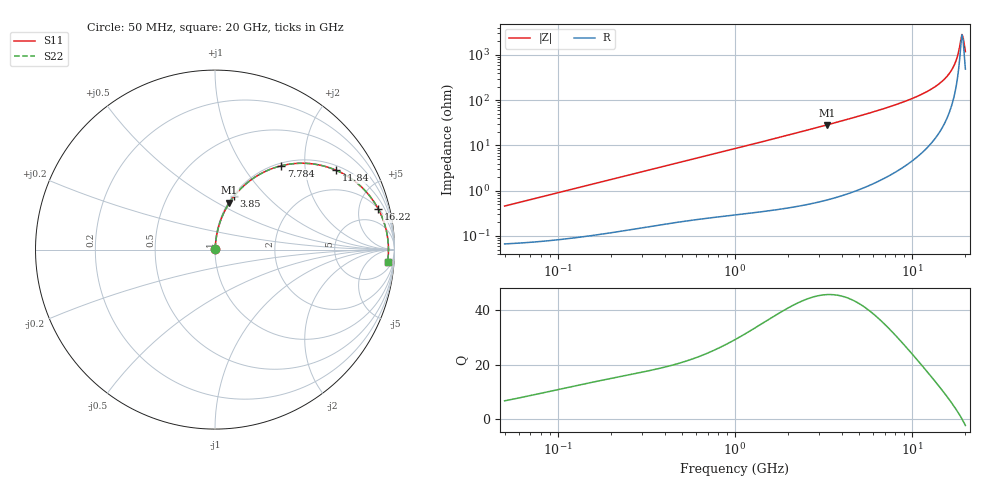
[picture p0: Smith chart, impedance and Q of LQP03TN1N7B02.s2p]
!Murata Part Number: LQP03TN1N7B02
!These Parameters are Measured in Series Mode Connection
!  o--[Z]--o
!Port1  Port2
!  o-------o
!Freq. Start=50[MHz] Stop=20[GHz], 401[Steps]
# Hz S RI R 50
!Freq.(Hz) S11(Real) S11(Imag) S21(Real) S21(Imag) S12(Real) S12(Imag) S22(Real) S22(Imag)
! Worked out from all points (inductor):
!   401 points, 50 MHz to 20 GHz, reference 50 ohm
!   read as one part in series: L = 1.44 nH near 51.52 MHz
!   highest Q = 45.6 at 3.314 GHz (marker M1), where L = 1.37 nH
!   self-resonance near 19.12 GHz
!   S11 on the Smith chart (normalised r, x): 50 MHz: 1.00, +0.01; 3.85 GHz: 1.01, +0.67; 7.784 GHz: 1.05, +1.51; 11.84 GHz: 1.16, +2.94; 16.22 GHz: 2.06, +7.70; 20 GHz: 11, -22
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5e7  0.00069 0.00454  0.9993 -0.00454  0.9993 -0.00454  0.00069 0.00454
1.364002e8  0.0011 0.0122  0.9989 -0.0122  0.9989 -0.0122  0.0011 0.0122
3.721004e8  0.00278 0.0323  0.9972 -0.0323  0.9972 -0.0323  0.00278 0.0323
1e9  0.0101 0.0841  0.9899 -0.0841  0.9899 -0.0841  0.0101 0.0841
2.728004e9  0.0561 0.2193  0.9439 -0.2193  0.9439 -0.2193  0.0561 0.2193
3.314454e9  0.0804 0.2612  0.9196 -0.2612  0.9196 -0.2612  0.0804 0.2612
3.850025e9  0.106 0.297  0.894 -0.297  0.894 -0.297  0.106 0.297
5.433528e9  0.1987 0.3869  0.8013 -0.3869  0.8013 -0.3869  0.1987 0.3869
7.442007e9  0.3423 0.4596  0.6577 -0.4596  0.6577 -0.4596  0.3423 0.4596
7.784049e9  0.3685 0.4669  0.6315 -0.4669  0.6315 -0.4669  0.3685 0.4669
9.745021e9  0.521 0.4798  0.479 -0.4798  0.479 -0.4798  0.521 0.4798
1.183995e10  0.6758 0.4416  0.3242 -0.4416  0.3242 -0.4416  0.6758 0.4416
1.417136e10  0.8199 0.3454  0.1801 -0.3454  0.1801 -0.3454  0.8199 0.3454
1.527346e10  0.8735 0.2838  0.1265 -0.2838  0.1265 -0.2838  0.8735 0.2838
1.621653e10  0.9107 0.2243  0.0893 -0.2243  0.0893 -0.2243  0.9107 0.2243
1.696185e10  0.934 0.1732  0.066 -0.1732  0.066 -0.1732  0.934 0.1732
1.747767e10  0.9467 0.1358  0.0533 -0.1358  0.0533 -0.1358  0.9467 0.1358
1.800918e10  0.9567 0.0956  0.0433 -0.0956  0.0433 -0.0956  0.9567 0.0956
1.88369e10  0.9655 0.0295  0.0345 -0.0295  0.0345 -0.0295  0.9655 0.0295
1.912117e10  0.9664 0.00574  0.0336 -0.00574  0.0336 -0.00574  0.9664 0.00574
1.940974e10  0.9661 -0.019  0.0339 0.019  0.0339 0.019  0.9661 -0.019
2e10  0.9612 -0.0714  0.0388 0.0714  0.0388 0.0714  0.9612 -0.0714
